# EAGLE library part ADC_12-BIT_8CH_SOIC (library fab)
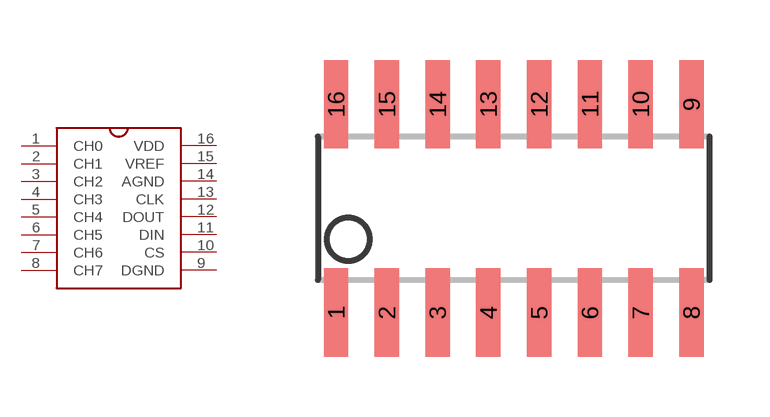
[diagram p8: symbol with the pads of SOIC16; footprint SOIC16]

Designator prefix -

## ADC_12-BIT_8CH_SOIC  [SOIC16]
1  CH0
2  CH1
3  CH2
4  CH3
5  CH4
6  CH5
7  CH6
8  CH7
9  DGND
10  CS
11  DIN
12  DOUT
13  CLK
14  AGND
15  VREF
16  VDD

## Footprint SOIC16 (pad centres in mm)
smd 0.61 x 2.21: 1 -3.81,-2.603; 2 -2.54,-2.603; 3 -1.27,-2.603; 4 0,-2.603; 5 1.27,-2.603; 6 2.54,-2.603; 7 3.81,-2.603; 8 5.08,-2.603; 9 5.08,2.603; 10 3.81,2.603; 11 2.54,2.603; 12 1.27,2.603; 13 0,2.603; 14 -1.27,2.603; 15 -2.54,2.603; 16 -3.81,2.603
